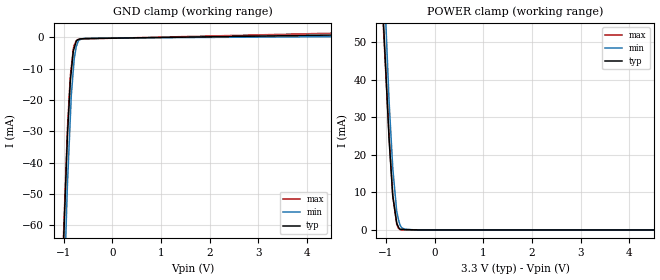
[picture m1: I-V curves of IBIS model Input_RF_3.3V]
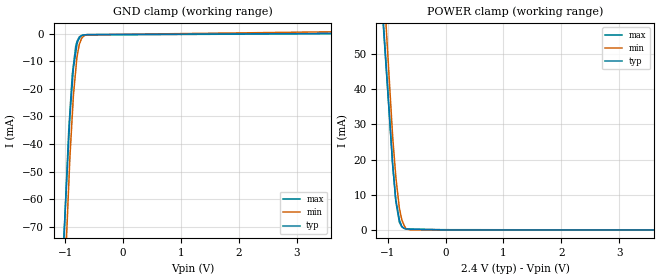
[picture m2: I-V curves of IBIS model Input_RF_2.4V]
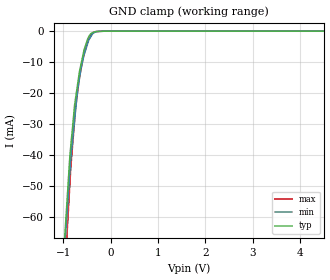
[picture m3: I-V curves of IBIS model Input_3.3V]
[IBIS Ver]   3.2
[Comment Char] |_char
[File Name]   pcm3008t.ibs
[File Rev]   3.0
[Source]
| This model file was created by Teraspeed Consulting Group LLC
| (http://www.teraspeed.com/).
[Date]   07-29-2004
[Notes]   Quality Check of this IBIS model: Model Passes IBIS Check
   Model parses into ICX IS. Simulation done with Hyperlynx.
   1. MIN TYP MAX information is based on Temprature and Voltage
   characteristics only.
[Disclaimer]
| This model is designed as an aid for customers of Texas Instruments.
| TI and its licensors and suppliers make no warranties, either expressed
| or implied, with respect to this  model, including the warranties of
| merchantability or fitness for a particular purpose.
| The model is provided solely on an "as is" basis. The entire risk as to
| its quality and performance is with the customer.
[Copyright]
| (C) Copyright 2008 Texas Instruments Incorporated. All rights reserved.
[Component] PCM3008T
[Manufacturer] TI
[Package]
| variable   typ   min   max
R_pkg  1.6023E-02  1.6023E-02  1.6023E-02
L_pkg  1.4421E-09  1.4421E-09  1.4421E-09
C_pkg  4.0058E-13  4.0058E-13  4.0058E-13
[Pin] signal_name  model_name  R_pin  L_pin C_pin
1   VCOM   POWER   1.7205E-02  1.5484E-09  4.3012E-13
2   VINR   Input_RF   1.6401E-02  1.4761E-09  4.1003E-13
3   VINL   Input_RF   1.5620E-02  1.4058E-09  3.9051E-13
4   GND   GND   1.4866E-02  1.3379E-09  3.7165E-13
5   VCC   POWER   1.4866E-02  1.3379E-09  3.7165E-13
6   DEM0   INPUT   1.5620E-02  1.4058E-09  3.9051E-13
7   DEM1   INPUT   1.6401E-02  1.4761E-09  4.1003E-13
8   DOUT   Output_DOUT  1.7205E-02  1.5484E-09  4.3012E-13
9   DIN   INPUT   1.7205E-02  1.5484E-09  4.3012E-13
10  LRCK   INPUT   1.6401E-02  1.4761E-09  4.1003E-13
11  SYSCK  INPUT   1.5620E-02  1.4058E-09  3.9051E-13
12  BCK   INPUT   1.4866E-02  1.3379E-09  3.7165E-13
13  _PDAD  INPUT   1.4866E-02  1.3379E-09  3.7165E-13
14  _PDDA  INPUT   1.5620E-02  1.4058E-09  3.9051E-13
15  VoutL  NC   1.6401E-02  1.4761E-09  4.1003E-13
16  VoutR  NC   1.7205E-02  1.5484E-09  4.3012E-13
[Model Selector] Input_RF
Input_RF_3.3V   Input at 3.3V with power clamp.
Input_RF_2.4V   Input at 2.4V with power clamp.
[Model Selector] INPUT
Input_3.3V   Input at 3.3V without power clamp.
Input_2.4V   Input at 2.4V without power clamp.
[Model Selector] Output_DOUT
Output_DOUT_3.3V  Output at 3.3V.
Output_DOUT_2.4V  Output at 2.4V.
| Models and submodels in the file (6): Input_RF_3.3V (Input), Input_RF_2.4V (Input), Input_3.3V (Input), Input_2.4V (Input), Output_DOUT_3.3V (Output), Output_DOUT_2.4V (Output)
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[Model] Input_RF_3.3V
Model_type Input
Vinl  = 990.000mV
Vinh  = 2.31000V
C_comp  1.57000pF 1.57000pF 1.57000pF
[Model Spec]
Vinh  2.3100V  2.1000V  2.5200V
Vinl  0.9900V  0.9000V  1.0800V
| variable   typ   min   max
[Voltage Range]   3.30000V  3.00000V  3.60000V
[POWER Clamp Reference]  3.30000V  3.00000V  3.60000V
[GND Clamp Reference]   0.00000V  0.00000V  0.00000V
[Temperature Range]   25   85   -25
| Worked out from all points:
|   GND clamp passes 1 mA (typ) near -0.72 V on its own axis
|   POWER clamp passes 1 mA (typ) near -0.75 V on its own axis
[GND Clamp]
-3.3V     -1.049A    -1.247A    -1.038A
-921.5mV  -31.84mA   -47.34mA   -29.55mA
-861.1mV  -13.93mA   -25.66mA   -12.29mA
-840.9mV  -10.77mA   -18.39mA   -9.455mA
-800.4mV  -4.465mA   -10.61mA   -3.781mA
-780.2mV  -3.396mA   -6.724mA   -2.424mA
-739.6mV  -1.257mA   -3.007mA   -1.14mA
-699.4mV  -764.4uA   -1.325mA   -693.3uA
-679.1mV  -621uA     -913.7uA   -632.4uA
-623.6mV  -495.6uA   -517uA     -566.2uA
-405.8mV  -388.1uA   -285.7uA   -464.4uA
6.6V      1.157mA    400.1uA    2.038mA
[POWER Clamp]
-3.3V     662.2mA    770.6mA    606.7mA
-1.059V   56.89mA    72.02mA    54.93mA
-1.019V   45.92mA    59.37mA    44.93mA
-958.7mV  29.74mA    40.69mA    30.18mA
-937.9mV  24.12mA    34.21mA    25.06mA
-862.1mV  9.069mA    16.38mA    8.982mA
-781.3mV  1.893mA    4.97mA     1.552mA
-740.8mV  587.3uA    2.522mA    342.6uA
-710.5mV  180.1uA    1.24mA     56.99uA
-609.2mV  90.47uA    179.4uA    0A
-402mV    38.43uA    2.479uA    0A
6.6V      0A         0A         0A
[Model] Input_RF_2.4V
Model_type Input
Vinl  = 720.000mV
Vinh  = 1.68000V
C_comp  1.57000pF 1.57000pF 1.57000pF
[Model Spec]
Vinh  1.6800V  1.4700V  1.8900V
Vinl  0.7200V  0.6300V  0.8100V
| variable   typ   min   max
[Voltage Range]   2.40000V  2.10000V  2.70000V
[POWER Clamp Reference]  2.40000V  2.10000V  2.70000V
[GND Clamp Reference]   0.00000V  0.00000V  0.00000V
[Temperature Range]   25   85   -25
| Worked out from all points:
|   GND clamp passes 1 mA (typ) near -0.74 V on its own axis
|   POWER clamp passes 1 mA (typ) near -0.76 V on its own axis
[GND Clamp]
-2.4V     -652.9mA   -779.9mA   -721.5mA
-942mV    -38.48mA   -54.78mA   -35.08mA
-921.5mV  -29.88mA   -44.63mA   -28.32mA
-881mV    -18.28mA   -29.67mA   -14.87mA
-861.1mV  -12.61mA   -22.36mA   -11.45mA
-820.7mV  -6.839mA   -13.17mA   -4.483mA
-800.4mV  -3.938mA   -8.547mA   -2.788mA
-780.2mV  -2.457mA   -6.225mA   -1.967mA
-759.9mV  -1.712mA   -3.893mA   -1.143mA
-719.4mV  -727.9uA   -1.651mA   -577.8uA
-620.9mV  -257.9uA   -339.5uA   -430.5uA
4.8V      209.5uA    1.025mA    213.1uA
[POWER Clamp]
-2.4V     393.9mA    438.1mA    378.8mA
-1.079V   59.39mA    71.34mA    57.98mA
-1.039V   49.31mA    60.29mA    48.31mA
-978.6mV  33.97mA    43.46mA    33.6mA
-917.4mV  18.47mA    26.47mA    18.73mA
-862.9mV  8.634mA    15.15mA    8.105mA
-801.8mV  2.959mA    6.229mA    2.221mA
-760.9mV  1.073mA    3.007mA    914.2uA
-720.7mV  446.6uA    1.356mA    479.7uA
-660.3mV  271.1uA    198.3uA    283.5uA
-539.1mV  158.8uA    13.59uA    231uA
4.8V      0A         0A         0A
[Model] Input_3.3V
Model_type Input
Vinl  = 990.000mV
Vinh  = 2.31000V
C_comp  1.57000pF 1.57000pF 1.57000pF
[Model Spec]
Vinh  2.3100V  2.1000V  2.5200V
Vinl  0.9900V  0.9000V  1.0800V
| variable   typ   min   max
[Voltage Range]   3.30000V  3.00000V  3.60000V
[POWER Clamp Reference]  3.30000V  3.00000V  3.60000V
[GND Clamp Reference]   0.00000V  0.00000V  0.00000V
[Temperature Range]   25   85   -25
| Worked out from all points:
|   GND clamp passes 1 mA (typ) near -0.43 V on its own axis
[GND Clamp]
-3.3V     -631.4mA   -585.9mA   -707.9mA
-861.2mV  -40.25mA   -45.51mA   -49.35mA
-840.9mV  -36.93mA   -41.03mA   -43.89mA
-759.9mV  -23.65mA   -28.54mA   -28.5mA
-739.8mV  -21.53mA   -25.43mA   -24.67mA
-699.5mV  -17.29mA   -19.21mA   -19.82mA
-658.9mV  -13.02mA   -15.27mA   -14.94mA
-562.3mV  -6.038mA   -7.661mA   -7.579mA
-481.7mV  -2.285mA   -3.774mA   -3.132mA
-400.7mV  -526.3uA   -1.277mA   -799.9uA
-90.25mV  42.35uA    83.83uA    90.77uA
6.6V      54.8uA     83.83uA    90.77uA
[POWER Clamp]
| Voltage   I(typ)   I(min)   I(max)
-3.6V     0A         0A         0A
-3.5V     0A         0A         0A
-3.4V     0A         0A         0A
7.2V      0A         0A         0A
